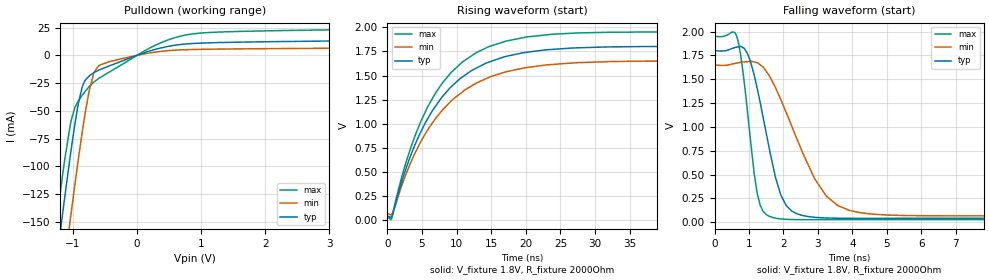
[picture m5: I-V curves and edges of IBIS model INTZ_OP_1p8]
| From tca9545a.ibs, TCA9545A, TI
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|   Model
[Model]   INTZ_OP_1p8
Model_type   Open_drain
Polarity   Non-Inverting
Vmeas = 0.9
Vref = 1.8
Cref = 1pF
Rref = 2000
|   typ   min   max
C_comp   1.601pF   1.487pF   1.862pF
[Voltage Range]   1.8   1.65   1.95
[Temperature Range]   27   125   -40
[Pullup Reference]   1.8   1.65   1.95
[Pulldown Reference]   -0   -0   -0
[Power Clamp Reference]   1.8   1.65   1.95
[GND Clamp Reference]   -0   -0   -0
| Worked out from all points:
|   slope of the pulldown table from 0 to 0.27 V, typ, clamps not added: 53 ohm
|   falling waveform, V_fixture 1.8V, R_fixture 2000Ohm: 20-80 % time 623ps typ, 1.17ns min, 364ps max; typ from 1.8 V to 0.041 V
|   rising waveform, V_fixture 1.8V, R_fixture 2000Ohm: 20-80 % time 8.16ns typ, 8.68ns min, 7.78ns max; typ from 0.041 V to 1.8 V
[Pulldown]
|   Voltage   I(typ)   I(min)   I(max)
-1.8V     -445.1mA   -504.7mA   -408mA
-1.26V    -187.5mA   -247.4mA   -151mA
-1.195V   -157.8mA   -217.4mA   -122.1mA
-1.163V   -143.1mA   -202.5mA   -108.1mA
-1.039V   -89mA      -146.3mA   -61.46mA
-925.2mV  -46.27mA   -97.34mA   -41.91mA
-860.4mV  -29.54mA   -71.13mA   -36.33mA
-741.6mV  -18.27mA   -30.47mA   -27.84mA
-595.8mV  -13.31mA   -9.18mA    -20.68mA
241.2mV   4.638mA    2.539mA    7.803mA
781.2mV   10.29mA    5.086mA    18.48mA
3.595V    13.22mA    6.593mA    23.44mA
[Ramp]
R_load = 2000
|   typ   min   max
dV/dt_r   1.05517/8.15835e-09   0.949544/8.68576e-09   1.15373/7.7822e-09
dV/dt_f   1.0552/6.22998e-10   0.949571/1.17473e-09   1.15375/3.63668e-10
[Falling Waveform]
V_fixture = 1.8V
V_fixture_min = 1.65V
V_fixture_max = 1.95V
R_fixture = 2000Ohm
C_fixture = 0F
|   Time   V(typ)   V(min)   V(max)
0s        1.8V       1.65V      1.95V
639ps     1.837V     1.67V      1.956V
954.6ps   1.771V     1.685V     1.162V
1.148ns   1.547V     1.682V     518mV
1.322ns   1.259V     1.652V     180.3mV
1.769ns   469.7mV    1.412V     43.12mV
2.106ns   166.5mV    1.128V     30.08mV
3.237ns   45.17mV    277.8mV    27.23mV
4.992ns   41.41mV    76.31mV    27.3mV
100ns     41.34mV    67.38mV    27.09mV
[Rising Waveform]
V_fixture = 1.8V
V_fixture_min = 1.65V
V_fixture_max = 1.95V
R_fixture = 2000Ohm
C_fixture = 0F
|   Time   V(typ)   V(min)   V(max)
0s        41.34mV    67.38mV    27.09mV
586.1ps   36.14mV    62.12mV    14.81mV
2.106ns   409.3mV    367mV      456.8mV
3.343ns   667.2mV    593.6mV    746.5mV
4.811ns   914.1mV    812.9mV    1.022V
6.892ns   1.176V     1.049V     1.312V
10.81ns   1.484V     1.33V      1.639V
17.12ns   1.698V     1.538V     1.856V
32.5ns    1.797V     1.645V     1.948V
100ns     1.8V       1.65V      1.95V
